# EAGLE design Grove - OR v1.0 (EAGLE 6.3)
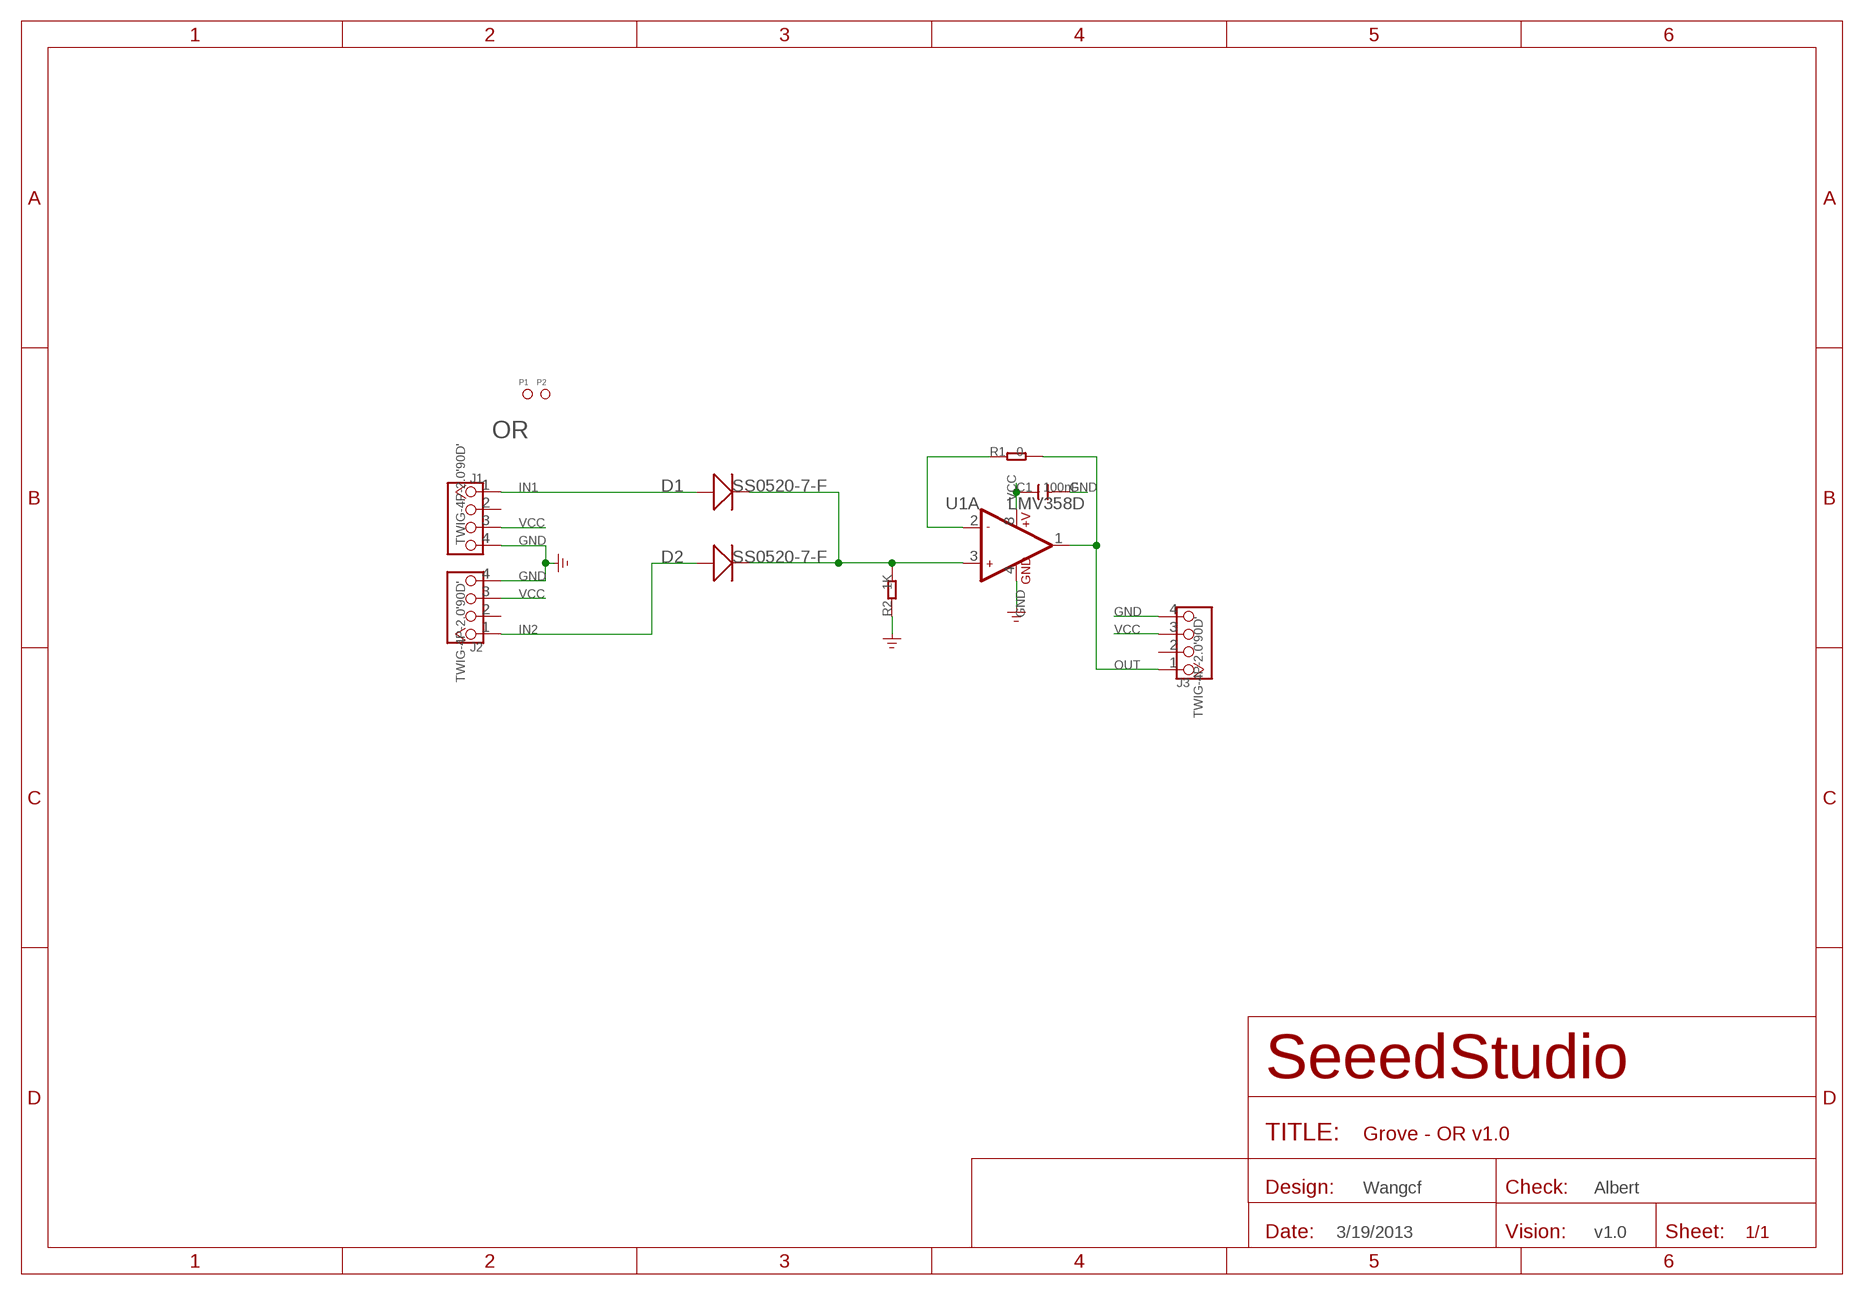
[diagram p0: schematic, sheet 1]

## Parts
C1  100nF  C-0603  [C0603]
D1  SS0520-7-F  D'1206'  [SOD123]
D2  SS0520-7-F  D'1206'  [SOD123]
J1  TWIG-4P-2.0'90D'  [4P-2.0-90D]
J2  TWIG-4P-2.0'90D'  [4P-2.0-90D]
J3  TWIG-4P-2.0'90D'  [4P-2.0-90D]
P1  PAD-MARK  [ROUND-MARK-1.0]
P2  PAD-MARK  [ROUND-MARK-1.0]
R1  0  R-0603  [R0603]
R2  1K  R-0603  [R0603]
U1  LMV358D  [SO08]

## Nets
GND: C1.2 J1.4 J2.4 J3.4 R2.1 U1.4(A:GND)
IN1: D1.+ J1.1
IN2: D2.+ J2.1
N$1: R1.1 U1.2(A:-IN1)
N$2: D1.- D2.- R2.2 U1.3(A:+IN1)
OUT: J3.1 R1.2 U1.1(A:OUT1)
VCC: C1.1 J1.3 J2.3 J3.3 U1.8(A:+V)
Unconnected: J1.2 J2.2 J3.2 U1.5(B:+IN2) U1.6(B:-IN2) U1.7(B:OUT2)

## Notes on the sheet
- OR
- Wangcf | Albert
- 3/19/2013 | v1.0

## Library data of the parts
C1 = Discrete:C*: Ceramic Capacitors
D1 D2 = Discrete:D*
J1-J3 = Connector:TWIG-4P-2.0
P1 P2 = Discrete:PAD-MARK; PARTNO: DNP
R1 R2 = Discrete:R*
U1 = IC:LMV358: General purpose LOW Voltage, Rail-to-Rail Output Amplifiers http://www.fairchildsemi.com/ds/LM/LMV358.pdf

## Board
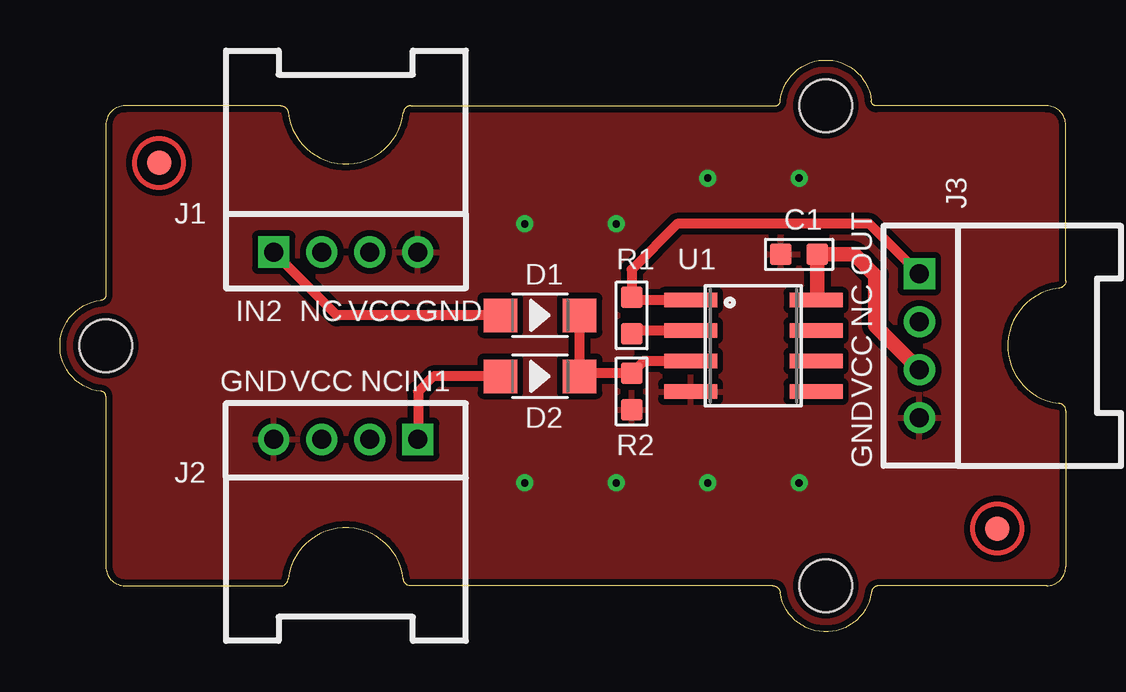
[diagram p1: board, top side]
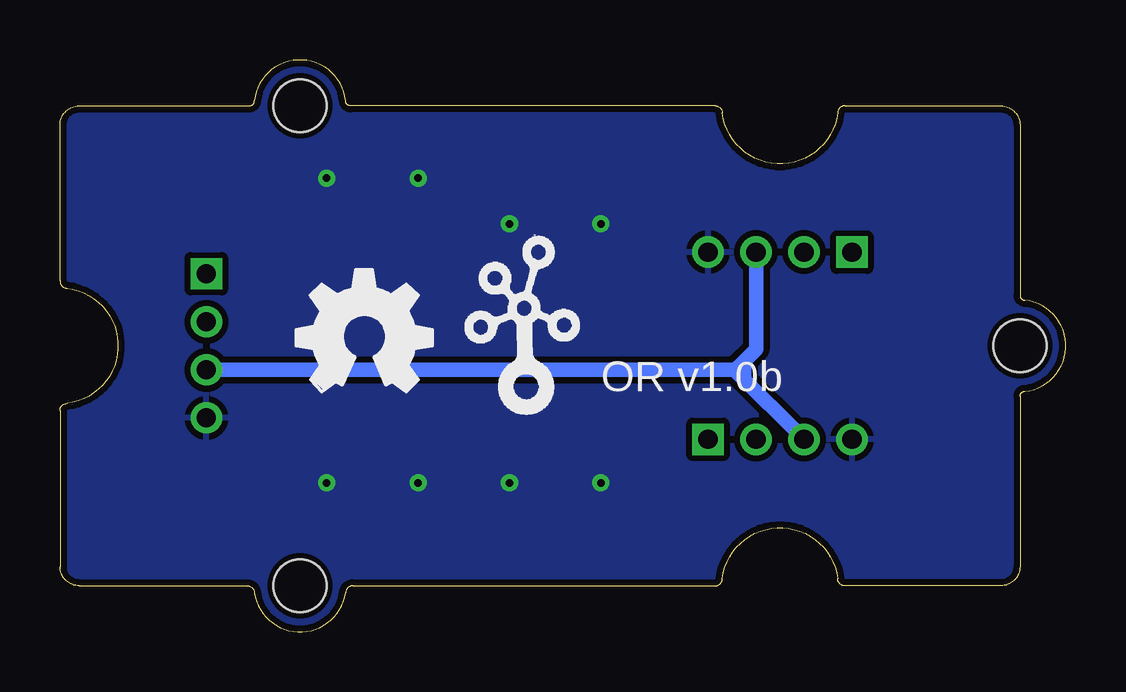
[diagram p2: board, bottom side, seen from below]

Size 41.91 x 23.83 mm. Coordinates in mm from the lower left corner, seen from the top.
Copper layers (1*16): Top 0.035mm / dielectric 1.5mm / Bottom 0.035mm
Design rules "default *": minimum track width 10mil, minimum drill 12mil, track to track 6mil, track to pad 6mil, pad to pad 6mil, via to via 6mil, smd to smd 0mil, copper to edge 10mil, drill to drill 8mil, minimum pad ring 10mil, minimum via ring 8mil, stop-mask expansion 4mil, vias tented up to drill 25mil, thermal gap 10mil

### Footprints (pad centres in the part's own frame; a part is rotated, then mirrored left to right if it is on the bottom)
C0603 = smd 0.889 x 0.889: 1 -0.762,0; 2 0.762,0
SOD123 = smd 1.397 x 1.397: + -1.651,0; - 1.651,0
4P-2.0-90D = drill 0.8 pad 1.27 square: 1 -3,0 | drill 0.8 pad 1.27: 2 -1,0; 3 1,0; 4 3,0
ROUND-MARK-1.0 = smd 1.016 x 1.016: P$1 0,0
R0603 = smd 0.889 x 0.889: 1 -0.762,0; 2 0.762,0
SO08 = smd 0.61 x 2.21: 1 -1.905,-2.616; 2 -0.635,-2.616; 3 0.635,-2.616; 4 1.905,-2.616; 5 1.905,2.616; 6 0.635,2.616; 7 -0.635,2.616; 8 -1.905,2.616
2U-DIM-W/DRILL = hole 2.2: -10,-10; -10,10; 20,0

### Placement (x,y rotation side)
C1  30.8,15.73 180 top
D1  20,13.19 0 top
D2  20,10.65 0 top
J1  11.91,15.82 0 top
J2  11.91,8.02 180 top
J3  35.81,11.92 270 top
P1  4.13,19.54 0 top
P2  39.05,4.3 0 top
R1  23.81,13.19 90 top
R2  23.81,10.02 90 top
U1  28.89,11.92 270 top
U$1  [2U-DIM-W/DRILL]  21.91,11.92 180 top
U$2  [OSHW_FILLX200_NOTEXT]  32.07,10.02 0 bottom
U$3  [TWIGLOGO]  22.54,10.02 0 bottom

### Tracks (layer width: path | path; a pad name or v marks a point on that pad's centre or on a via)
GND  (via drill 0.3 pad 0.64)
  other vias: 19.37,6.21 23.18,6.21 26.99,6.21 19.37,17 23.18,17 30.8,6.21 26.99,18.91 30.8,18.91
  pour Bottom (isolate 0.254): -0.32,23.99 42.86,23.99 42.86,-0.14 -0.32,-0.14
  pour Top (isolate 0.254): -0.32,23.99 42.86,23.99 42.86,-0.14 -0.32,-0.14
IN1
  Top 0.406: D1.+ 11.54,13.19 J1.1
IN2
  Top 0.406: D2.+ 15.56,10.65 14.92,10.02 14.92,8.04 J2.1
N$1
  Top 0.406: U1.2 23.94,12.56 R1.1
N$2
  Top 0.406: U1.3 24.32,11.29 R2.2 21.78,10.78 D2.- D1.-
OUT
  Top 0.406: U1.1 23.94,13.83 R1.2 23.81,15.1 25.72,17 33.72,17 J3.1
VCC
  Top 0.61: U1.8 31.56,13.88 C1.1 33.08,15.73 33.97,14.84 33.97,12.76 J3.3
  Bottom 0.61: J3.3 13.81,10.92 13.79,10.9 | 13.79,10.9 J2.3 | J1.3 12.91,11.78 13.4,11.29 | 13.4,11.29 13.79,10.9 | 13.4,11.29 13.4,10.52

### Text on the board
tPlace: OUT | IN2 | NC | VCC | GND | NC | GND | VCC | NC | IN1 | VCC | GND
bPlace: OR v1.0b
